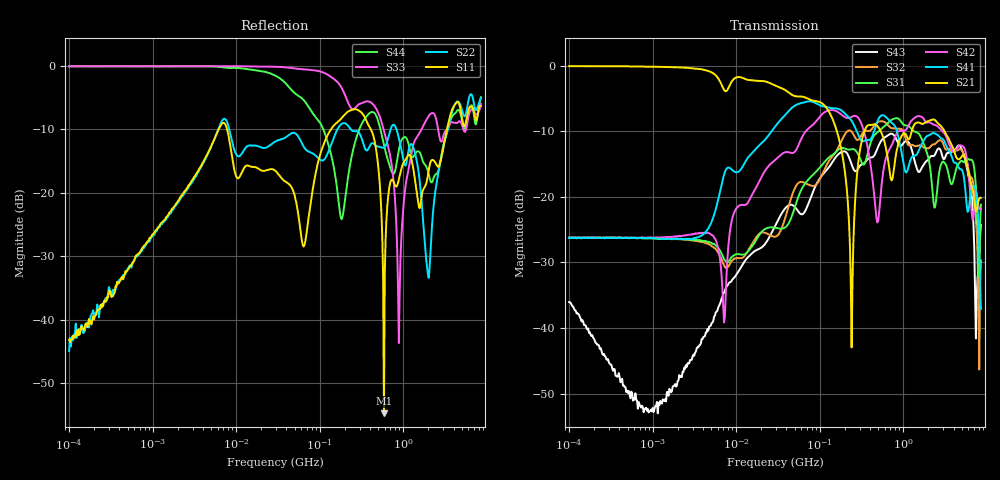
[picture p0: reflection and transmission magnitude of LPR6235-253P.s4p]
# MHz S MA R 50
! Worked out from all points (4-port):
!   498 points, 100 kHz to 8.5 GHz, reference 50 ohm
!   strongest paths, dB at 100 kHz, 1.698 MHz, 29.49 MHz, 500.7 MHz, 8.5 GHz:
!     S21: -0.1, -0.2, -3.1, -9.3, -20.2
!     S41: -26.3, -26.4, -9.2, -8.2, -37.1
!     S42: -26.3, -26.1, -14.3, -23.7, -21.9
!     S31: -26.3, -26.4, -24.7, -10.1, -21.2
!     S32: -26.2, -26.5, -26.1, -8.6, -29.7
!     S43: -36.1, -49.7, -24.3, -12.4, -24.3
!   lowest |S11| = -54.8 dB at 587.5 MHz (marker M1), VSWR 1.00, Z = 50.2 - j0.045 ohm
!   |S11| at or under -10 dB: start of sweep to 6.195 MHz; 7.773 MHz to 136.7 MHz (128.9 MHz wide, 178 % of centre); 408.8 MHz to 3.338 GHz (2.929 GHz wide, 156 % of centre)
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0.1  0.00695 38.5  0.9901 -0.3  0.04865 -178.9  0.04869 2.2
     0.9901 -0.3  0.005647 47.8  0.04891 1.1  0.04869 179.4
     0.04865 -178.9  0.04891 1.1  0.9897 0.8  0.01576 -79.2
     0.04869 2.2  0.04869 179.4  0.01576 -79.2  0.9904 0.8
6.995403  0.3551 8.2  0.6717 -19.0  0.03474 148.2  0.1396 74.1
          0.6717 -19.0  0.3788 30.1  0.03107 -6.2  0.01475 83.8
          0.03474 148.2  0.03107 -6.2  0.9918 -2.8  0.0181 83.7
          0.1396 74.1  0.01475 83.8  0.0181 83.7  0.9692 -10.9
317.0858  0.4263 -70.7  0.2638 -0.1  0.1834 -13.9  0.2672 -58.7
          0.2638 -0.1  0.2689 -68.2  0.2964 -14.0  0.3581 -77.7
          0.1834 -13.9  0.2964 -14.0  0.5065 -78.7  0.1766 -15.6
          0.2672 -58.7  0.3581 -77.7  0.1766 -15.6  0.3463 -6.1
587.4518  0.001828 -14.2  0.2717 -97.6  0.3426 -52.2  0.4161 -89.8
          0.2717 -97.6  0.2262 -98.0  0.3733 -72.7  0.1684 -38.4
          0.3426 -52.2  0.3733 -72.7  0.3081 -158.9  0.2811 -55.7
          0.4161 -89.8  0.1684 -38.4  0.2811 -55.7  0.2389 -115.1
886.1403  0.1268 -111.3  0.2605 -91.1  0.3918 -118.9  0.275 -156.1
          0.2605 -91.1  0.2692 174.1  0.3303 -122.6  0.3166 -95.5
          0.3918 -118.9  0.3303 -122.6  0.006536 -155.1  0.2511 -118.2
          0.275 -156.1  0.3166 -95.5  0.2511 -118.2  0.2167 -113.5
1970.81  0.1362 132.7  0.3768 102.3  0.2053 55.0  0.2924 103.7
         0.3768 102.3  0.02299 -42.8  0.2341 100.4  0.3683 89.0
         0.2053 55.0  0.2341 100.4  0.3925 114.5  0.1912 112.8
         0.2924 103.7  0.3683 89.0  0.1912 112.8  0.1493 81.7
8500  0.4802 -26.8  0.09798 44.9  0.08716 -4.2  0.01395 -61.0
      0.09798 44.9  0.5558 -43.2  0.03272 0.6  0.0801 -29.2
      0.08716 -4.2  0.03272 0.6  0.4998 -14.0  0.06093 26.3
      0.01395 -61.0  0.0801 -29.2  0.06093 26.3  0.565 -39.8
